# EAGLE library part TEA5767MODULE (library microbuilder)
TEA5767 FM-Receiver Module - 87.5-108MHz
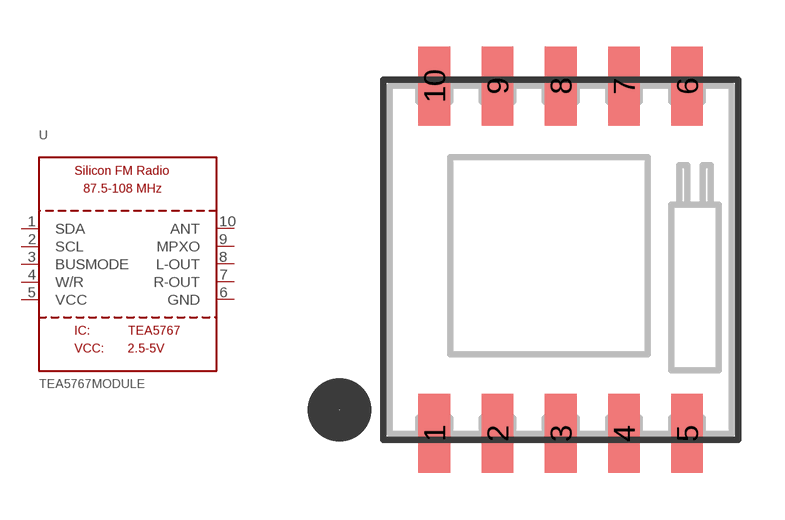
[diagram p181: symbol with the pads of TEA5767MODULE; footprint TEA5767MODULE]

Designator prefix U

## TEA5767MODULE  [TEA5767MODULE]
1  SDA
2  SCL
3  BUSMODE
4  W/R
5  VCC
6  GND
7  R-OUT
8  L-OUT
9  MPXO
10  ANT

## Footprint TEA5767MODULE (pad centres in mm)
smd 1.016 x 2.54: 1 -4.064,-5.588; 2 -2.032,-5.588; 3 0,-5.588; 4 2.032,-5.588; 5 4.064,-5.588; 6 4.064,5.588; 7 2.032,5.588; 8 0,5.588; 9 -2.032,5.588; 10 -4.064,5.588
